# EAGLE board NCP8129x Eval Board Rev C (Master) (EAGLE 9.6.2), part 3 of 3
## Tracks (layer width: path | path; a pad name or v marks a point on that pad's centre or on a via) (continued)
VOUT  (via drill 0.15 pad 0.3) (continued)
  other vias: 37.43,64.48 37.83,64.48 37.03,64.48 38.23,64.48 38.63,64.48 39.03,64.48 39.43,64.48 39.83,64.48 39.63,64.83 39.23,64.83 38.83,64.83 38.43,64.83 38.03,64.83 37.63,64.83 37.23,64.83 36.83,64.83 39.83,65.18 39.43,65.18 39.03,65.18 38.63,65.18 38.23,65.18 37.83,65.18 37.43,65.18 37.03,65.18 36.63,65.18 36.83,65.53 36.43,65.53 37.23,65.53 37.63,65.53 38.03,65.53 38.43,65.53 38.83,65.53 39.23,65.53 39.63,65.53 40.03,65.53 36.63,65.88 36.23,65.88 37.03,65.88 37.43,65.88 37.83,65.88 38.23,65.88 38.63,65.88 39.03,65.88 39.43,65.88 39.83,65.88 40.23,65.88 35.78,76.48 35.38,76.48 34.98,76.48 34.58,76.48 34.18,76.48 33.78,76.48 33.38,76.48 32.98,76.48 32.58,76.48 32.18,76.48 35.58,76.18 35.18,76.18 34.78,76.18 34.38,76.18 33.98,76.18 33.58,76.18 33.18,76.18 32.38,76.18 32.78,76.18 31.98,76.18 35.98,76.18 32.18,75.88 32.58,75.88 32.98,75.88 33.38,75.88 33.78,75.88 34.18,75.88 34.58,75.88 34.98,75.88 35.38,75.88 35.78,75.88 31.98,75.58 32.38,75.58 32.78,75.58 33.18,75.58 33.58,75.58 33.98,75.58 34.38,75.58 34.78,75.58 35.18,75.58 35.58,75.58 35.98,75.58 32.18,75.28 32.58,75.28 32.98,75.28 33.38,75.28 33.78,75.28 34.18,75.28 34.58,75.28 34.98,75.28 35.38,75.28 35.78,75.28 31.98,74.98 32.38,74.98 32.78,74.98 33.18,74.98 33.58,74.98 33.98,74.98 34.38,74.98 34.78,74.98 35.18,74.98 35.58,74.98 35.98,74.98 35.78,74.68 35.38,74.68 34.98,74.68 34.58,74.68 34.18,74.68 32.18,74.68 32.58,74.68 32.98,74.68 33.38,74.68 33.78,74.68 45.08,76.48 44.68,76.48 44.28,76.48 43.88,76.48 43.48,76.48 43.08,76.48 42.68,76.48 42.28,76.48 41.88,76.48 41.48,76.48 44.88,76.18 44.48,76.18 44.08,76.18 43.68,76.18 43.28,76.18 42.88,76.18 42.48,76.18 41.68,76.18 42.08,76.18 41.28,76.18 45.28,76.18 41.48,75.88 41.88,75.88 42.28,75.88 42.68,75.88 43.08,75.88 43.48,75.88 43.88,75.88 44.28,75.88 44.68,75.88 45.08,75.88 41.28,75.58 41.68,75.58 42.08,75.58 42.48,75.58 42.88,75.58 43.28,75.58 43.68,75.58 44.08,75.58 44.48,75.58 44.88,75.58 45.28,75.58 41.48,75.28 41.88,75.28 42.28,75.28 42.68,75.28 43.08,75.28 43.48,75.28 43.88,75.28 44.28,75.28 44.68,75.28 45.08,75.28 41.28,74.98 41.68,74.98 42.08,74.98 42.48,74.98 42.88,74.98 43.28,74.98 43.68,74.98 44.08,74.98 44.48,74.98 44.88,74.98 45.28,74.98 45.08,74.68 44.68,74.68 44.28,74.68 43.88,74.68 43.48,74.68 41.48,74.68 41.88,74.68 42.28,74.68 42.68,74.68 43.08,74.68 36.13,69.18 35.73,69.18 35.33,69.18 35.53,68.88 35.93,68.88 35.33,68.58 35.73,68.58 36.13,68.58 35.53,68.28 35.93,68.28 35.33,67.98 35.73,67.98 36.13,67.98 41.93,69.18 41.53,69.18 41.13,69.18 41.33,68.88 41.73,68.88 41.13,68.58 41.53,68.58 41.93,68.58 41.33,68.28 41.73,68.28 41.13,67.98 41.53,67.98 41.93,67.98 41.33,69.48 41.73,69.48 42.13,69.48 40.93,69.48 41.13,69.78 41.53,69.78 41.93,69.78 42.33,69.78 40.93,68.88 40.93,68.28 41.33,70.08 40.93,70.08 41.73,70.08 42.13,70.08 42.53,70.08 42.73,69.78 42.93,70.08 43.13,69.78 43.33,70.08 43.53,69.78 43.73,70.08 41.13,70.38 40.73,70.38 40.73,69.78 40.73,69.18 40.73,68.58 40.73,67.98 41.53,70.38 41.93,70.38 42.33,70.38 43.93,69.78 44.13,70.08 44.33,69.78 44.53,70.08 44.73,69.78 44.93,70.08 44.53,69.48 44.93,69.48 44.73,69.18 44.53,68.88 44.93,68.88 44.73,68.58 44.53,68.28 42.73,70.38 43.13,70.38 43.53,70.38 43.93,70.38 44.33,70.38 44.73,70.38 40.93,70.68 41.33,70.68 41.73,70.68 42.13,70.68 42.53,70.68 42.93,70.68 43.33,70.68 43.73,70.68 44.13,70.68 44.53,70.68 44.93,70.68 40.73,70.98 41.13,70.98 41.53,70.98 41.93,70.98 42.33,70.98 42.73,70.98 43.13,70.98 43.53,70.98 43.93,70.98 44.33,70.98 44.73,70.98 40.93,71.28 41.33,71.28 41.73,71.28 42.13,71.28 42.53,71.28 44.53,71.28 44.13,71.28 43.73,71.28 43.33,71.28 42.93,71.28 44.93,71.28 44.73,71.58 44.33,71.58 43.93,71.58 43.53,71.58 43.13,71.58 42.73,71.58 42.33,71.58 41.93,71.58 41.53,71.58 41.13,71.58 40.73,71.58 40.93,71.88 41.33,71.88 41.73,71.88 42.13,71.88 42.53,71.88 42.93,71.88 43.33,71.88 43.73,71.88 44.13,71.88 44.53,71.88 44.93,71.88 40.73,72.18 41.13,72.18 41.53,72.18 41.93,72.18 44.73,72.18 44.33,72.18 43.93,72.18 43.53,72.18 43.13,72.18 42.73,72.18 42.33,72.18 36.63,67.83 37.43,67.83 38.23,67.83 39.03,67.83 39.83,67.83 37.03,68.23 37.83,68.23 38.63,68.23 39.43,68.23 40.23,68.23 39.83,68.63 39.03,68.63 38.23,68.63 37.43,68.63 36.63,68.63 37.03,69.03 37.83,69.03 38.63,69.03 39.43,69.03 40.23,69.03 39.83,69.43 39.03,69.43 38.23,69.43 37.43,69.43 36.63,69.43 37.03,69.83 37.83,69.83 38.63,69.83 39.43,69.83 40.23,69.83 36.23,69.83 35.43,69.83 35.83,70.23 36.63,70.23 37.43,70.23 38.23,70.23 39.03,70.23 39.83,70.23 40.23,70.63 39.43,70.63 38.63,70.63 37.83,70.63 37.03,70.63 36.23,70.63 35.43,70.63 39.83,71.03 39.03,71.03 38.23,71.03 37.43,71.03 36.63,71.03 35.83,71.03 35.43,71.43 36.23,71.43 37.03,71.43 37.83,71.43 38.63,71.43 39.43,71.43 40.23,71.43 39.83,71.83 39.03,71.83 38.23,71.83 37.43,71.83 36.63,71.83 35.83,71.83 35.03,71.83 35.43,72.23 36.23,72.23 37.03,72.23 37.83,72.23 38.63,72.23 39.43,72.23 40.23,72.23 34.63,72.23 35.03,72.63 35.83,72.63 36.63,72.63 37.43,72.63 38.23,72.63 39.03,72.63 39.83,72.63 40.63,72.63 41.43,72.63 42.23,72.63 43.03,72.63 43.83,72.63 44.63,72.63 34.23,72.63 34.63,73.03 35.43,73.03 36.23,73.03 37.03,73.03 37.83,73.03 38.63,73.03 39.43,73.03 40.23,73.03 41.03,73.03 41.83,73.03 42.63,73.03 43.43,73.03 44.23,73.03 45.03,73.03 33.83,73.03 33.43,73.43 34.23,73.43 35.03,73.43 35.83,73.43 44.63,73.43 43.83,73.43 43.03,73.43 42.23,73.43 41.43,73.43 40.63,73.43 39.83,73.43 39.03,73.43 38.23,73.43 37.43,73.43 36.63,73.43 33.03,73.83 33.83,73.83 34.63,73.83 35.43,73.83 36.23,73.83 37.03,73.83 37.83,73.83 38.63,73.83 39.43,73.83 40.23,73.83 41.03,73.83 41.83,73.83 42.63,73.83 43.43,73.83 44.23,73.83 45.03,73.83 44.63,74.23 43.83,74.23 43.03,74.23 42.23,74.23 41.43,74.23 40.63,74.23 39.83,74.23 39.03,74.23 38.23,74.23 37.43,74.23 36.63,74.23 35.83,74.23 35.03,74.23 34.23,74.23 33.43,74.23 32.63,74.23 36.23,74.63 37.03,74.63 37.83,74.63 38.63,74.63 39.43,74.63 40.23,74.63 41.03,74.63 40.63,75.03 39.83,75.03 39.03,75.03 38.23,75.03 37.43,75.03 36.63,75.03 37.03,75.43 37.83,75.43 38.63,75.43 39.43,75.43 40.23,75.43 40.63,75.83 39.83,75.83 39.03,75.83 38.23,75.83 37.43,75.83 36.63,75.83 37.03,76.23 37.83,76.23 38.63,76.23 39.43,76.23 40.23,76.23 36.63,76.63 37.43,76.63 38.23,76.63 39.03,76.63 39.83,76.63 40.63,76.63 37.03,77.03 36.23,77.03 35.43,77.03 34.63,77.03 33.83,77.03 33.03,77.03 32.23,77.03 37.83,77.03 38.63,77.03 39.43,77.03 40.23,77.03 41.03,77.03 41.83,77.03 42.63,77.03 43.43,77.03 44.23,77.03 45.03,77.03 32.63,77.43 33.43,77.43 34.23,77.43 35.03,77.43 35.83,77.43 36.63,77.43 37.43,77.43 38.23,77.43 39.03,77.43 39.83,77.43 40.63,77.43 41.43,77.43 42.23,77.43 43.03,77.43 43.83,77.43 44.63,77.43 45.03,77.83 44.23,77.83 43.43,77.83 42.63,77.83 41.83,77.83 41.03,77.83 40.23,77.83 39.43,77.83 38.63,77.83 37.83,77.83 37.03,77.83 36.23,77.83 35.43,77.83 34.63,77.83 33.83,77.83 33.03,77.83 32.23,77.83 44.63,78.23 45.03,78.63 44.63,79.03 44.23,78.63 44.23,79.43 43.83,78.23 43.83,79.03 43.83,79.83 43.43,78.63 43.43,79.43 43.43,80.23 43.03,78.23 43.03,79.03 43.03,79.83 43.03,80.63 42.63,78.63 42.63,79.43 42.63,80.23 42.63,81.03 42.23,78.23 42.23,79.03 42.23,79.83 42.23,80.63 42.23,81.43 41.83,78.63 41.83,79.43 41.83,80.23 41.83,81.03 41.83,81.83 41.43,78.23 41.43,79.03 41.43,79.83 41.43,80.63 41.43,81.43 41.43,82.23 41.03,78.63 41.03,79.43 41.03,80.23 41.03,81.03 41.03,81.83 40.63,78.23 40.63,79.03 40.63,79.83 40.63,80.63 40.63,81.43 40.63,82.23 40.63,83.03 41.03,82.63 40.23,78.63 40.23,79.43 40.23,80.23 40.23,81.03 40.23,81.83 40.23,82.63 40.23,83.43 39.83,78.23 39.83,79.03 39.83,79.83 39.83,80.63 39.83,81.43 39.83,82.23 39.83,83.03 39.83,83.83 39.43,78.63 39.43,79.43 39.43,80.23 39.43,81.03 39.43,81.83 39.43,82.63 39.43,83.43 39.43,84.23 39.03,78.23 39.03,79.03 39.03,79.83 39.03,80.63 39.03,81.43 39.03,82.23 39.03,83.03 39.03,83.83 39.03,84.63 38.23,78.23 38.63,78.63 38.63,79.43 38.63,80.23 38.63,81.03 38.63,81.83 38.63,82.63 38.63,83.43 38.63,84.23 38.63,85.03 38.23,79.03 38.23,79.83 38.23,80.63 38.23,81.43 38.23,82.23 38.23,83.03 38.23,83.83 38.23,84.63 38.23,85.43 37.83,78.63 37.83,79.43 37.83,80.23 37.83,81.03 37.83,81.83 37.83,82.63 37.83,83.43 37.83,84.23 37.83,85.03 37.83,85.83 37.43,78.23 37.43,79.03 37.43,79.83 37.43,80.63 37.43,81.43 37.43,82.23 37.43,83.03 37.43,83.83 37.43,84.63 37.43,85.43 37.43,86.23 37.03,78.63 37.03,79.43 37.03,80.23 37.03,81.03 37.03,81.83 37.03,82.63 37.03,83.43 37.03,84.23 37.03,85.03 37.03,85.83 37.03,86.63 36.63,78.23 36.63,79.03 36.63,79.83 36.63,80.63 36.63,81.43 36.63,82.23 36.63,83.03 36.63,83.83 36.63,84.63 36.63,85.43 36.63,86.23 36.63,87.03 36.23,78.63 36.23,79.43 36.23,80.23 36.23,81.03 36.23,81.83 36.23,82.63 36.23,83.43 36.23,84.23 36.23,85.03 36.23,85.83 36.23,86.63 36.23,87.43 35.83,78.23 35.83,79.03 35.83,79.83 35.83,80.63 35.83,81.43 35.83,82.23 35.83,83.03 35.83,83.83 35.83,84.63 35.83,85.43 35.83,86.23 35.83,87.03 35.83,87.83 35.43,78.63 35.43,79.43 35.43,80.23 35.43,81.03 35.43,81.83 35.43,82.63 35.43,83.43 35.43,84.23 35.43,85.03 35.43,85.83 35.43,86.63 35.43,87.43 35.43,88.23 35.03,78.23 35.03,79.03 35.03,79.83 35.03,80.63 35.03,88.63 35.03,87.83 35.03,87.03 35.03,86.23 35.03,85.43 35.03,84.63 35.03,83.83 35.03,83.03 35.03,82.23 35.03,81.43 34.63,78.63 34.63,79.43 34.63,80.23 34.63,81.03 34.63,81.83 34.63,82.63 34.63,83.43 34.63,84.23 34.63,85.03 34.63,85.83 34.63,86.63 34.63,87.43 34.63,88.23 34.63,89.03 34.23,78.23 34.23,79.03 34.23,79.83 34.23,80.63 34.23,81.43 34.23,82.23 34.23,83.03 34.23,83.83 34.23,84.63 34.23,85.43 34.23,86.23 34.23,87.03 34.23,87.83 34.23,88.63 34.23,89.43 33.83,78.63 33.83,79.43 33.83,80.23 33.83,81.03 33.83,81.83 33.83,82.63 33.83,83.43 33.83,84.23 33.83,85.03 33.83,85.83 33.83,86.63 33.83,87.43 33.83,88.23 33.83,89.03 33.83,89.83 33.43,78.23 33.43,79.03 33.43,79.83 33.43,80.63 33.43,81.43 33.43,82.23 33.43,83.03 33.43,83.83 33.43,84.63 33.43,85.43 33.43,86.23 33.43,87.03 33.43,87.83 33.43,88.63 33.43,89.43 33.43,90.23 33.03,78.63 33.03,79.43 33.03,80.23 33.03,81.03 33.03,81.83 33.03,82.63 33.03,83.43 33.03,84.23 33.03,85.03 33.03,85.83 33.03,86.63 33.03,87.43 33.03,88.23 33.03,89.03 33.03,89.83 33.03,90.63 32.63,78.23 32.63,79.03 32.63,79.83 32.63,80.63 32.63,81.43 32.63,82.23 32.63,83.03 32.63,83.83 32.63,84.63 32.63,85.43 32.63,86.23 32.63,87.03 32.63,87.83 32.63,88.63 32.63,89.43 32.63,90.23 32.63,91.03 32.23,78.63 32.23,79.43 32.23,80.23 32.23,81.03 32.23,81.83 32.23,82.63 32.23,83.43 32.23,84.23 32.23,85.03 32.23,85.83 32.23,86.63 32.23,87.43 32.23,88.23 32.23,89.03 32.23,89.83 32.23,90.63 32.23,91.43 45.03,84.23 44.63,84.63 44.23,85.03 43.83,85.43 43.43,85.83 43.03,86.23 42.63,86.63 42.23,87.03 41.83,87.43 41.43,87.83 41.03,88.23 40.63,88.63 40.23,89.03 39.83,89.43 39.43,89.83 39.03,90.23 38.63,90.63 38.23,91.03 37.83,91.43 37.43,91.83 37.03,92.23 36.63,92.63 36.23,93.03 35.83,93.43 35.43,93.83 35.03,94.23 34.63,94.63 34.23,95.03 33.83,95.43 33.43,95.83 33.03,96.23 32.63,96.63 32.23,97.03 45.03,85.03 44.63,85.43 44.23,85.83 43.83,86.23 43.43,86.63 43.03,87.03 42.63,87.43 42.23,87.83 41.83,88.23 41.43,88.63 41.03,89.03 40.63,89.43 40.23,89.83 39.83,90.23 39.43,90.63 39.03,91.03 38.63,91.43 38.23,91.83 37.83,92.23 37.43,92.63 37.03,93.03 36.63,93.43 36.23,93.83 35.83,94.23 35.43,94.63 35.03,95.03 34.63,95.43 34.23,95.83 33.83,96.23 33.43,96.63 33.03,97.03 32.63,97.43 32.23,97.83 45.43,84.63 45.83,85.03 46.23,85.43 45.83,85.83 45.43,85.43 45.03,85.83 45.43,86.23 45.03,86.63 44.63,86.23 44.23,86.63 44.63,87.03 44.23,87.43 43.83,87.03 43.43,87.43 43.83,87.83 43.43,88.23 43.03,87.83 42.63,88.23 43.03,88.63 42.63,89.03 42.23,88.63 42.23,89.43 41.83,89.03 41.43,89.43 41.83,89.83 41.43,90.23 41.03,89.83 40.63,90.23 41.03,90.63 40.63,91.03 40.23,90.63 39.83,91.03 40.23,91.43 39.83,91.83 39.43,91.43 39.03,91.83 39.43,92.23 39.03,92.63 38.63,92.23 38.23,92.63 38.63,93.03 38.23,93.43 37.83,93.03 37.43,93.43 37.83,93.83 37.43,94.23 37.03,93.83 36.63,94.23 37.03,94.63 36.63,95.03 36.23,94.63 35.83,95.03 36.23,95.43 35.83,95.83 35.43,95.43 35.03,95.83 35.43,96.23 35.03,96.63 34.63,96.23 34.23,96.63 34.63,97.03 33.83,97.03 34.23,97.43 33.43,97.43 33.83,97.83 33.03,97.83 33.43,98.23 33.03,98.63 32.63,98.23 46.63,85.83 47.03,86.23 47.43,86.63 47.03,87.03 46.63,86.63 46.23,86.23 45.83,86.63 46.23,87.03 46.63,87.43 46.23,87.83 45.83,87.43 45.43,87.03 45.03,87.43 45.43,87.83 45.83,88.23 45.43,88.63 45.03,88.23 44.63,87.83 44.23,88.23 44.63,88.63 45.03,89.03 44.63,89.43 44.23,89.03 43.83,88.63 43.43,89.03 43.83,89.43 44.23,89.83 43.03,89.43 43.43,89.83 43.83,90.23 43.43,90.63 43.03,90.23 42.63,89.83 42.23,90.23 42.63,90.63 43.03,91.03 41.83,90.63 42.23,91.03 42.63,91.43 42.23,91.83 41.83,91.43 41.43,91.03 41.03,91.43 41.43,91.83 41.83,92.23 41.43,92.63 41.03,92.23 40.63,91.83 40.23,92.23 40.63,92.63 41.03,93.03 40.63,93.43 40.23,93.03 39.83,92.63 39.43,93.03 39.83,93.43 40.23,93.83 39.83,94.23 39.43,93.83 39.03,93.43 38.63,93.83 39.03,94.23 39.43,94.63 39.03,95.03 38.63,94.63 38.23,94.23 37.83,94.63 38.23,95.03 38.63,95.43 37.43,95.03 37.83,95.43 38.23,95.83 37.83,96.23 37.43,95.83 37.03,95.43 36.63,95.83 37.03,96.23 37.43,96.63 37.03,97.03 36.63,96.63 36.23,96.23 35.83,96.63 36.23,97.03 36.63,97.43 36.23,97.83 35.83,97.43 35.43,97.03 35.03,97.43 35.43,97.83 35.83,98.23 35.43,98.63 35.03,98.23 34.63,97.83 34.23,98.23 34.63,98.63 35.03,99.03 34.63,99.43 34.23,99.03 33.83,98.63 33.43,99.03 33.83,99.43 34.23,99.83 47.83,87.03 48.23,87.43 47.43,87.43 47.83,87.83 48.23,88.23 47.03,87.83 47.43,88.23 47.83,88.63 48.23,89.03 46.63,88.23 47.03,88.63 47.43,89.03 47.83,89.43 48.23,89.83 46.23,88.63 46.63,89.03 47.03,89.43 47.43,89.83 47.83,90.23 48.23,90.63 45.83,89.03 46.23,89.43 46.63,89.83 47.03,90.23 47.43,90.63 47.83,91.03 48.23,91.43 45.43,89.43 45.83,89.83 46.23,90.23 46.63,90.63 47.03,91.03 47.43,91.43 47.83,91.83 48.23,92.23 45.03,89.83 45.43,90.23 45.83,90.63 46.23,91.03 46.63,91.43 47.03,91.83 47.43,92.23 47.83,92.63 48.23,93.03 44.63,90.23 45.03,90.63 45.43,91.03 45.83,91.43 46.23,91.83 46.63,92.23 47.03,92.63 47.43,93.03 47.83,93.43 48.23,93.83 44.23,90.63 44.63,91.03 45.03,91.43 45.43,91.83 45.83,92.23 46.23,92.63 46.63,93.03 47.03,93.43 47.43,93.83 47.83,94.23 48.23,94.63 43.83,91.03 44.23,91.43 44.63,91.83 45.03,92.23 45.43,92.63 45.83,93.03 46.23,93.43 46.63,93.83 47.03,94.23 47.43,94.63 47.83,95.03 48.23,95.43 43.43,91.43 43.83,91.83 44.23,92.23 44.63,92.63 45.03,93.03 45.43,93.43 45.83,93.83 46.23,94.23 46.63,94.63 47.03,95.03 47.43,95.43 47.83,95.83 48.23,96.23 43.03,91.83 43.43,92.23 43.83,92.63 44.23,93.03 44.63,93.43 45.03,93.83 45.43,94.23 45.83,94.63 46.23,95.03 46.63,95.43 47.03,95.83 47.43,96.23 47.83,96.63 48.23,97.03 42.63,92.23 43.03,92.63 43.43,93.03 43.83,93.43 44.23,93.83 44.63,94.23 45.03,94.63 45.43,95.03 45.83,95.43 46.23,95.83 46.63,96.23 47.03,96.63 47.43,97.03 47.83,97.43 48.23,97.83 42.23,92.63 42.63,93.03 43.03,93.43 43.43,93.83 43.83,94.23 44.23,94.63 44.63,95.03 45.03,95.43 45.43,95.83 46.23,96.63 45.83,96.23 46.63,97.03 47.03,97.43 47.43,97.83 47.83,98.23 48.23,98.63 41.83,93.03 42.23,93.43 42.63,93.83 43.03,94.23 43.43,94.63 43.83,95.03 44.23,95.43 44.63,95.83 45.03,96.23 45.43,96.63 45.83,97.03 46.23,97.43 46.63,97.83 47.03,98.23 47.43,98.63 47.83,99.03 48.23,99.43 41.43,93.43 41.83,93.83 42.23,94.23 42.63,94.63 43.03,95.03 43.43,95.43 43.83,95.83 44.23,96.23 44.63,96.63 45.03,97.03 45.43,97.43 45.83,97.83 46.23,98.23 46.63,98.63 47.03,99.03 47.43,99.43 47.83,99.83 48.23,100.23 41.03,93.83 41.43,94.23 41.83,94.63 42.23,95.03 42.63,95.43 43.03,95.83 43.43,96.23 43.83,96.63 44.23,97.03 44.63,97.43 45.03,97.83 45.43,98.23 45.83,98.63 46.23,99.03 46.63,99.43 47.03,99.83 47.43,100.23 47.83,100.63 48.23,101.03 40.63,94.23 41.03,94.63 41.43,95.03 41.83,95.43 42.23,95.83 42.63,96.23 43.03,96.63 43.43,97.03 43.83,97.43 44.23,97.83 44.63,98.23 45.03,98.63 45.43,99.03 45.83,99.43 46.23,99.83 46.63,100.23 47.03,100.63 47.43,101.03 47.83,101.43 48.23,101.83 40.23,94.63 40.63,95.03 41.03,95.43 41.43,95.83 41.83,96.23 42.23,96.63 42.63,97.03 43.03,97.43 43.43,97.83 43.83,98.23 44.23,98.63 44.63,99.03 45.03,99.43 45.43,99.83 45.83,100.23 46.23,100.63 46.63,101.03 47.03,101.43 47.43,101.83 47.83,102.23 48.23,102.63 39.83,95.03 40.23,95.43 40.63,95.83 41.03,96.23 41.43,96.63 41.83,97.03 42.23,97.43 42.63,97.83 43.03,98.23 43.43,98.63 43.83,99.03 44.23,99.43 44.63,99.83 45.03,100.23 45.43,100.63 45.83,101.03 46.23,101.43 46.63,101.83 47.03,102.23 47.43,102.63 47.83,103.03 48.23,103.43 39.43,95.43 39.83,95.83 40.23,96.23 40.63,96.63 41.03,97.03 41.43,97.43 41.83,97.83 42.23,98.23 42.63,98.63 43.03,99.03 43.43,99.43 43.83,99.83 44.23,100.23 44.63,100.63 45.03,101.03 45.43,101.43 45.83,101.83 46.23,102.23 46.63,102.63 47.03,103.03 47.43,103.43 47.83,103.83 48.23,104.23 39.03,95.83 39.43,96.23 39.83,96.63 40.23,97.03 40.63,97.43 41.03,97.83 41.43,98.23 41.83,98.63 42.23,99.03 42.63,99.43 43.03,99.83 43.43,100.23 43.83,100.63 44.23,101.03 44.63,101.43 45.03,101.83 45.43,102.23 45.83,102.63 46.23,103.03 46.63,103.43 47.03,103.83 47.43,104.23 47.83,104.63 48.23,105.03 38.63,96.23 39.03,96.63 39.43,97.03 39.83,97.43 40.23,97.83 40.63,98.23 41.03,98.63 41.43,99.03 41.83,99.43 42.23,99.83 42.63,100.23 43.03,100.63 43.43,101.03 43.83,101.43 44.23,101.83 44.63,102.23 45.03,102.63 45.43,103.03 45.83,103.43 46.23,103.83 46.63,104.23 47.03,104.63 47.43,105.03 47.83,105.43 48.23,105.83 38.23,96.63 38.63,97.03 39.03,97.43 39.43,97.83 39.83,98.23 40.23,98.63 40.63,99.03 41.03,99.43 41.43,99.83 41.83,100.23 42.23,100.63 42.63,101.03 43.03,101.43 43.43,101.83 43.83,102.23 44.23,102.63 44.63,103.03 45.03,103.43 45.43,103.83 45.83,104.23 46.23,104.63 46.63,105.03 47.03,105.43 47.43,105.83 47.83,106.23 48.23,106.63 37.83,97.03 38.23,97.43 38.63,97.83 39.03,98.23 39.43,98.63 39.83,99.03 40.23,99.43 40.63,99.83 41.03,100.23 41.43,100.63 41.83,101.03 42.23,101.43 42.63,101.83 43.03,102.23 43.43,102.63 43.83,103.03 44.23,103.43 44.63,103.83 45.03,104.23 45.43,104.63 45.83,105.03 46.23,105.43 46.63,105.83 47.03,106.23 47.43,106.63 47.83,107.03 48.23,107.43 37.43,97.43 37.83,97.83 38.23,98.23 38.63,98.63 39.03,99.03 39.43,99.43 39.83,99.83 40.23,100.23 40.63,100.63 41.03,101.03 41.43,101.43 41.83,101.83 42.23,102.23 42.63,102.63 43.03,103.03 43.43,103.43 43.83,103.83 44.23,104.23 44.63,104.63 45.03,105.03 45.43,105.43 45.83,105.83 46.23,106.23 46.63,106.63 47.03,107.03 47.43,107.43 47.83,107.83 48.23,108.23 37.03,97.83 37.43,98.23 37.83,98.63 38.23,99.03 38.63,99.43 39.03,99.83 39.43,100.23 39.83,100.63 40.23,101.03 40.63,101.43 41.03,101.83 41.43,102.23 41.83,102.63 42.23,103.03 42.63,103.43 43.03,103.83 43.43,104.23 43.83,104.63 44.23,105.03 44.63,105.43 45.03,105.83 45.43,106.23 45.83,106.63 46.23,107.03 46.63,107.43 47.03,107.83 47.43,108.23 47.83,108.63 48.23,109.03 36.63,98.23 37.03,98.63 37.43,99.03 37.83,99.43 38.23,99.83 38.63,100.23 39.03,100.63 39.43,101.03 39.83,101.43 40.23,101.83 40.63,102.23 41.03,102.63 41.43,103.03 41.83,103.43 42.23,103.83 42.63,104.23 43.03,104.63 43.43,105.03 43.83,105.43 44.23,105.83 44.63,106.23 45.03,106.63 45.43,107.03 45.83,107.43 46.23,107.83 46.63,108.23 47.03,108.63 47.43,109.03 47.83,109.43 48.23,109.83 36.23,98.63 36.63,99.03 37.03,99.43 37.43,99.83 37.83,100.23 38.23,100.63 38.63,101.03 39.03,101.43 39.43,101.83 39.83,102.23 40.23,102.63 40.63,103.03 41.03,103.43 41.43,103.83 41.83,104.23 42.23,104.63 42.63,105.03 43.03,105.43 43.43,105.83 43.83,106.23 44.23,106.63 44.63,107.03 45.03,107.43 45.43,107.83 45.83,108.23 46.23,108.63 46.63,109.03 47.03,109.43 47.43,109.83 47.83,110.23 35.83,99.03 36.23,99.43 36.63,99.83 37.03,100.23 37.43,100.63 37.83,101.03 38.23,101.43 38.63,101.83 39.03,102.23 39.43,102.63 39.83,103.03 40.23,103.43 40.63,103.83 41.03,104.23 41.43,104.63 41.83,105.03 42.23,105.43 42.63,105.83 43.03,106.23 43.43,106.63 43.83,107.03 44.23,107.43 44.63,107.83 45.03,108.23 45.43,108.63 45.83,109.03 46.23,109.43 46.63,109.83 47.03,110.23 35.43,99.43 35.83,99.83 36.23,100.23 36.63,100.63 37.03,101.03 37.43,101.43 37.83,101.83 38.23,102.23 38.63,102.63 39.03,103.03 39.43,103.43 39.83,103.83 40.23,104.23 40.63,104.63 41.03,105.03 41.43,105.43 41.83,105.83 42.23,106.23 42.63,106.63 43.03,107.03 43.43,107.43 43.83,107.83 44.23,108.23 44.63,108.63 45.03,109.03 45.43,109.43 45.83,109.83 46.23,110.23 35.03,99.83 35.43,100.23 35.83,100.63 36.23,101.03 36.63,101.43 37.03,101.83 37.43,102.23 37.83,102.63 38.23,103.03 38.63,103.43 39.03,103.83 39.43,104.23 39.83,104.63 40.23,105.03 40.63,105.43 41.03,105.83 41.43,106.23 41.83,106.63 42.23,107.03 42.63,107.43 43.03,107.83 43.43,108.23 43.83,108.63 44.23,109.03 44.63,109.43 45.03,109.83 45.43,110.23 34.63,100.23 35.03,100.63 35.43,101.03 35.83,101.43 36.23,101.83 36.63,102.23 37.03,102.63 37.43,103.03 37.83,103.43 38.23,103.83 38.63,104.23 39.03,104.63 39.43,105.03 39.83,105.43 40.23,105.83 40.63,106.23 41.03,106.63 41.43,107.03 41.83,107.43 42.23,107.83 42.63,108.23 43.03,108.63 43.43,109.03 43.83,109.43 44.23,109.83 44.63,110.23 43.83,110.23 44.23,110.63 43.83,111.03 44.23,111.43 44.63,111.03 43.83,111.83 44.23,112.23 43.83,112.63 44.23,113.03 43.83,113.43 44.23,113.83 43.83,114.23 44.23,114.63 43.83,115.03 44.23,115.43 43.83,115.83 44.23,116.23 43.83,116.63 44.23,117.03 43.83,117.43 44.23,117.83 43.83,118.23 44.23,118.63 43.83,119.03 44.23,119.43 43.83,119.83 44.23,120.23 43.83,120.63 44.23,121.03 43.83,121.43 44.63,111.83 44.63,112.63 44.63,113.43 44.63,114.23 44.63,115.03 44.63,115.83 44.63,116.63 44.63,117.43 44.63,118.23 44.63,119.03 44.63,119.83 44.63,120.63 44.63,121.43 45.43,121.43 46.23,121.43 47.03,121.43 47.83,121.43 48.63,121.43 49.43,121.43 50.23,121.43 51.03,121.43 51.83,121.43 52.63,121.43 53.43,121.43 54.23,121.43 45.03,121.03 45.83,121.03 46.63,121.03 47.43,121.03 48.23,121.03 49.03,121.03 49.83,121.03 50.63,121.03 51.43,121.03 52.23,121.03 53.03,121.03 53.83,121.03 54.23,120.63 53.43,120.63 53.83,120.23 53.03,120.23 53.43,119.83 54.23,119.83 52.63,120.63 53.83,119.43 53.03,119.43 53.43,119.03 54.23,119.03 53.83,118.63 53.03,118.63 53.43,118.23 54.23,118.23 53.03,117.83 53.83,117.83 53.43,117.43 54.23,117.43 53.03,117.03 53.83,117.03 53.43,116.63 54.23,116.63 53.03,116.23 53.83,116.23 53.43,115.83 54.23,115.83 53.03,115.43 53.83,115.43 53.43,115.03 54.23,115.03 53.03,114.63 53.83,114.63 53.43,114.23 54.23,114.23 53.03,113.83 53.83,113.83 53.43,113.43 54.23,113.43 53.03,113.03 53.83,113.03 53.43,112.63 54.23,112.63 53.83,112.23 53.03,112.23 53.43,111.83 54.23,111.83 53.03,111.43 53.83,111.43 48.63,110.23 49.43,110.23 50.23,110.23 51.03,110.23 51.83,110.23 52.63,110.23 53.43,110.23 54.23,110.23 53.43,111.03 54.23,111.03 53.03,110.63 53.83,110.63 49.03,109.83 49.83,109.83 50.63,109.83 51.43,109.83 52.23,109.83 53.03,109.83 53.83,109.83 54.23,109.43 53.43,109.43 52.63,109.43 51.83,109.43 51.03,109.43 50.23,109.43 49.43,109.43 48.63,109.43 49.03,109.03 49.83,109.03 50.63,109.03 51.43,109.03 52.23,109.03 53.03,109.03 53.83,109.03 54.23,108.63 53.43,108.63 52.63,108.63 51.83,108.63 51.03,108.63 50.23,108.63 49.43,108.63 48.63,108.63 49.03,108.23 49.83,108.23 50.63,108.23 51.43,108.23 52.23,108.23 53.03,108.23 53.83,108.23 54.23,107.83 53.43,107.83 52.63,107.83 51.83,107.83 51.03,107.83 50.23,107.83 49.43,107.83 48.63,107.83 49.03,107.43 49.83,107.43 50.63,107.43 51.43,107.43 52.23,107.43 53.03,107.43 53.83,107.43 48.63,107.03 49.43,107.03 50.23,107.03 51.03,107.03 51.83,107.03 52.63,107.03 53.43,107.03 54.23,107.03 49.03,106.63 49.83,106.63 50.63,106.63 51.43,106.63 52.23,106.63 53.03,106.63 53.83,106.63 54.63,106.63 48.63,106.23 49.43,106.23 50.23,106.23 51.03,106.23 51.83,106.23 52.63,106.23 53.43,106.23 54.23,106.23 55.03,106.23 49.03,105.83 49.83,105.83 50.63,105.83 51.43,105.83 52.23,105.83 53.03,105.83 53.83,105.83 54.63,105.83 55.43,105.83 48.63,105.43 49.43,105.43 50.23,105.43 51.03,105.43 51.83,105.43 52.63,105.43 53.43,105.43 54.23,105.43 55.03,105.43 55.83,105.43 49.03,105.03 49.83,105.03 50.63,105.03 51.43,105.03 52.23,105.03 53.03,105.03 53.83,105.03 54.63,105.03 55.43,105.03 56.23,105.03 48.63,104.63 49.43,104.63 50.23,104.63 51.03,104.63 51.83,104.63 52.63,104.63 53.43,104.63 54.23,104.63 55.03,104.63 55.83,104.63 56.63,104.63 49.03,104.23 49.83,104.23 50.63,104.23 51.43,104.23 52.23,104.23 53.03,104.23 53.83,104.23 54.63,104.23 55.43,104.23 56.23,104.23 57.03,104.23 48.63,103.83 49.43,103.83 50.23,103.83 51.03,103.83 51.83,103.83 52.63,103.83 53.43,103.83 54.23,103.83 55.03,103.83 55.83,103.83 56.63,103.83 57.43,103.83 49.03,103.43 49.83,103.43 50.63,103.43 51.43,103.43 52.23,103.43 53.03,103.43 53.83,103.43 54.63,103.43 55.43,103.43 56.23,103.43 57.03,103.43 57.83,103.43 48.63,103.03 49.43,103.03 50.23,103.03 51.03,103.03 51.83,103.03 52.63,103.03 53.43,103.03 54.23,103.03 55.03,103.03 55.83,103.03 56.63,103.03 57.43,103.03 58.23,103.03 49.03,102.63 49.83,102.63 50.63,102.63 51.43,102.63 52.23,102.63 53.03,102.63 53.83,102.63 54.63,102.63 55.43,102.63 56.23,102.63 57.03,102.63 57.83,102.63 58.63,102.63 48.63,102.23 49.43,102.23 50.23,102.23 51.03,102.23 51.83,102.23 52.63,102.23 53.43,102.23 54.23,102.23 55.03,102.23 55.83,102.23 56.63,102.23 57.43,102.23 58.23,102.23 59.03,102.23 49.03,101.83 49.83,101.83 50.63,101.83 51.43,101.83 52.23,101.83 53.03,101.83 53.83,101.83 54.63,101.83 55.43,101.83 56.23,101.83 57.03,101.83 57.83,101.83 58.63,101.83 59.43,101.83 48.63,101.43 49.43,101.43 50.23,101.43 51.03,101.43 51.83,101.43 52.63,101.43 53.43,101.43 54.23,101.43 55.03,101.43 55.83,101.43 56.63,101.43 57.43,101.43 58.23,101.43 59.03,101.43 59.83,101.43 49.03,101.03 49.83,101.03 50.63,101.03 51.43,101.03 52.23,101.03 53.03,101.03 53.83,101.03 54.63,101.03 55.43,101.03 56.23,101.03 57.03,101.03 57.83,101.03 58.63,101.03 59.43,101.03 60.23,101.03 48.63,100.63 49.43,100.63 50.23,100.63 51.03,100.63 51.83,100.63 52.63,100.63 53.43,100.63 54.23,100.63 55.03,100.63 55.83,100.63 56.63,100.63 57.43,100.63 58.23,100.63 59.03,100.63 59.83,100.63 60.63,100.63
  pour +5V (no thermals): 39.98,64.33 36.78,64.33 36.13,64.98 36.13,65.98 40.33,65.98 40.33,65.68 40.03,65.38 39.98,65.33
  pour GND (no thermals): 39.98,64.33 36.78,64.33 36.43,64.68 36.13,64.98 36.13,65.38 36.13,65.98 40.33,65.98 40.33,65.68 40.28,65.63 39.98,65.33
  pour Top (no thermals): 36.78,64.33 35.23,65.88 35.23,68.23 35.23,71.18 31.88,74.53 31.88,97.98 43.43,109.53 43.43,121.98 54.63,121.98 54.63,107.48 61.63,100.48 61.63,87.48 48.68,87.48 46.63,85.43 45.38,84.18 45.38,76.18 45.38,68.98 44.53,68.13 44.43,68.13 44.43,69.53 44.28,69.68 42.48,69.68 42.08,69.28 42.08,67.88 40.48,66.28 40.33,66.13 40.33,65.83 40.33,65.68 39.98,65.33 39.98,65.23 39.98,64.33
  pour Bottom (no thermals): 43.43,121.98 43.43,109.53 42.88,108.98 31.88,97.98 31.88,74.53 32.13,74.28 35.23,71.18 35.23,67.78 35.23,65.88 36.78,64.33 39.98,64.33 39.98,65.28 40.23,65.53 40.33,65.63 40.33,65.83 40.33,66.13 40.53,66.33 41.33,67.13 44.68,67.13 44.98,67.13 45.03,67.13 45.03,72.08 45.38,72.43 45.38,84.18 48.68,87.48 61.63,87.48 61.63,100.48 54.78,107.33 54.63,107.48 54.63,107.68 54.63,121.98
  pour Power/fusetofuse1 (isolate 0.3, no thermals): 39.98,64.33 -0.72,64.33 -0.72,124.43 75.43,124.43 75.43,64.33
  pour Power1 (isolate 0.3, no thermals): -0.72,124.43 -0.72,64.33 75.43,64.33 75.43,124.43
  pour Power/fusetoio1 (isolate 0.3, no thermals): -0.72,64.33 -0.72,124.43 75.43,124.43 75.43,64.33
  pour Power2 (isolate 0.3, no thermals): -0.72,64.33 -0.72,124.43 75.43,124.43 75.43,64.33
  pour Power/fusetoio2 (isolate 0.3, no thermals): -0.72,124.43 -0.72,64.33 75.43,64.33 75.43,124.43
  pour Power3 (isolate 0.3, no thermals): -0.72,124.43 -0.72,64.33 75.43,64.33 75.43,124.43
  pour Power/misc (isolate 0.3, no thermals): -0.72,64.33 -0.72,124.43 75.43,124.43 75.43,64.33
  pour Power4 (isolate 0.3, no thermals): -0.72,64.33 -0.72,124.43 75.43,124.43 75.43,64.33
  pour Top (no thermals): 36.53,63.38 35.73,63.38 35.53,63.58 35.23,63.88 35.23,65.93 36.88,65.93 36.88,64.33 36.58,64.33 36.53,64.33
  pour Bottom (no thermals): 40.73,63.38 41.48,63.38 45.03,66.93 45.03,67.18 40.78,67.18 39.98,66.38 39.98,65.63 40.83,65.63 40.83,64.18 40.73,64.08
VOUT_S  (via drill 0.15 pad 0.3)  (1 unrouted)
  Power/fusetoio1 0.3: IC1.25 40.38,65.08 42.43,67.13 44.78,67.13 45.48,67.83 45.48,72.68 47.58,74.78 47.58,85.08 48.53,86.03 62.53,86.03 63.03,86.53 63.03,112.73 v60.23,115.53
  other vias: 40.38,64.68
VTEMP  (via drill 0.15 pad 0.3)  (4 unrouted)
  Top 1: TP14.1 68.3,54.61 68.99,55.3 J5.2
  Power/fusetofuse1 0.3: v45.73,58.78 45.73,58.33 44.63,57.23 32.58,57.23 31.58,58.23 v31.58,58.78
  Power/misc 0.3: v45.73,58.78 46.63,58.78 50.83,54.58 v62.78,54.58
  other vias: 72.53,55.28
VTEMP1  (via drill 0.15 pad 0.3)  (2 unrouted)
  Top 0.3: IC1.18 42.98,60.98 43.33,60.63 43.33,59.68 43.96,59.05 R9.1
  Top 0.5: C15.1 44.28,59.03 R9.1
  Power/fusetoio1 0.3: v9.43,45.68 8.03,44.28 8.03,41.93 8.83,41.13 23.48,41.13 28.83,46.48 28.83,50.73 29.48,51.38 35.63,51.38 36.98,52.73 43.73,52.73 44.28,53.28 C15.1
  other vias: 44.28,57.78
VTEMP2  (via drill 0.15 pad 0.3)  (2 unrouted)
  Power/fusetoio2 0.3: v9.38,76.18 8.43,75.23 8.43,71.33 22.03,57.73 v32.98,57.73
  Bottom 0.3: R16.1 33.56,59.05 34.08,59.58 34.08,60.68 34.38,60.98 IC2.18
  Bottom 0.5: C18.1 32.98,59.03 R16.1

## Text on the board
tNames: GND | VOUT | ONSEMI NCP8129x / Modular Demo Board / "Master" Unit Rev C / SN: | GND | GND | ENABLE SW | OFF | BOTTOM IC | ON | GND | CLREF | CS | D_OC | IMON | VOUT CON | ON | VDD | GOK | NC1 | SS | VINF | GOK | VTEMP | ON | GATE | D_OC | TOP IC | IMON | CLREF | RESET | CS | D_OC | SS | IMON | ON | VTEMP | VDD | GOK | +5V | SS | GND | VINF | VTEMP | GND | GND | GATE | TP29 | TP30 | GND | VIN CON | D_OC | GOK | RESET SW | GND | VIN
